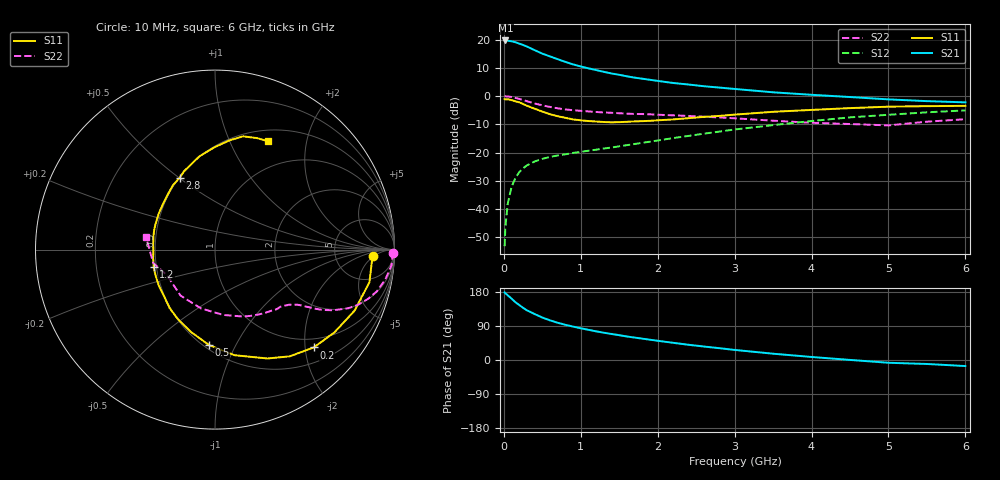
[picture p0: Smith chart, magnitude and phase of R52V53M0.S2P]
! SIEMENS Small Signal Semiconductors
! BFR183
! Si NPN RF Bipolar Junction Transistor in SOT23
! VCE = 2.5 V  IC = 3 mA
! Common Emitter S-Parameters:  May  1996
# GHz  S  MA  R  50
!  f  S11  S21  S12  S22
! GHz  MAG  ANG  MAG  ANG  MAG  ANG  MAG  ANG
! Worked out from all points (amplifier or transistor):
!   36 points, 10 MHz to 6 GHz, reference 50 ohm
!   highest |S21| = 19.7 dB at 20 MHz (marker M1)
!   |S21| within 3 dB of that: start of sweep to 366.3 MHz
!   unconditionally stable (mu >= 1): 1.244 GHz to 2.767 GHz
!   at 250 MHz: K = 0.30, MSG = 21.8 dB, |S12| = -25.5 dB
!   at 1.4 GHz: K = 1.05, MAG = 11.7 dB, |S12| = -18.2 dB
!   at 6 GHz: K = 0.90, MSG = 1.4 dB, |S12| = -5.1 dB
!   lowest NFmin = 1.10 dB at 450 MHz
!   S11 on the Smith chart (normalised r, x): 10 MHz: 14, -5; 200 MHz: 0.80, -2.18; 500 MHz: 0.53, -0.79; 1.2 GHz: 0.48, -0.11; 2.8 GHz: 0.50, +0.50; 6 GHz: 0.64, +1.41
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0.01  0.8822 -2.4  9.584 178.4  0.0022 89.9  0.9946 -1.0
0.02  0.8765 -4.5  9.675 176.1  0.0048 84.0  0.9897 -2.1
0.05  0.8793 -11.9  9.576 170.9  0.0123 83.4  0.9869 -5.1
0.1  0.8489 -23.6  9.343 162.0  0.0247 77.0  0.9637 -9.9
0.15  0.8094 -34.8  9.014 152.5  0.0353 71.5  0.931 -14.5
0.2  0.7747 -44.7  8.513 145.1  0.0449 67.1  0.8951 -17.9
0.25  0.726 -55.0  8.051 137.7  0.0528 62.4  0.8541 -21.1
0.3  0.6738 -64.2  7.55 131.1  0.0594 59.0  0.8122 -23.7
0.4  0.5982 -79.6  6.519 121.3  0.0695 54.3  0.742 -27.1
0.5  0.5328 -93.6  5.651 112.1  0.0775 51.0  0.6871 -29.3
0.6  0.4779 -106.3  5.047 104.6  0.0837 49.4  0.6432 -30.7
0.7  0.4401 -117.7  4.505 98.3  0.089 48.7  0.6084 -31.7
0.9  0.3867 -136.7  3.642 88.1  0.0986 48.3  0.5627 -33.3
1.1  0.3618 -155.9  3.103 79.7  0.1079 49.4  0.5356 -35.0
1.2  0.3551 -164.4  2.891 75.6  0.1125 49.9  0.5235 -35.9
1.6  0.351 167.7  2.243 62.0  0.1353 52.9  0.4893 -40.2
2.2  0.3861 138.4  1.708 45.4  0.1805 55.0  0.457 -49.2
2.8  0.4458 116.2  1.417 31.2  0.235 53.1  0.419 -61.8
3.5  0.5274 99.4  1.168 16.6  0.3064 47.3  0.3669 -82.8
4.5  0.613 82.6  0.963 0.2  0.4204 35.6  0.3203 -126.7
5.5  0.6642 69.2  0.815 -10.5  0.5165 21.9  0.3524 -167.8
6  0.6719 63.8  0.775 -16.0  0.5587 13.3  0.3899 169.8
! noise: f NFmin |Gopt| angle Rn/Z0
0.45  1.1  0.37  35  0.3
0.9  1.15  0.34  85  0.23
1.8  1.9  0.35  160  0.13
